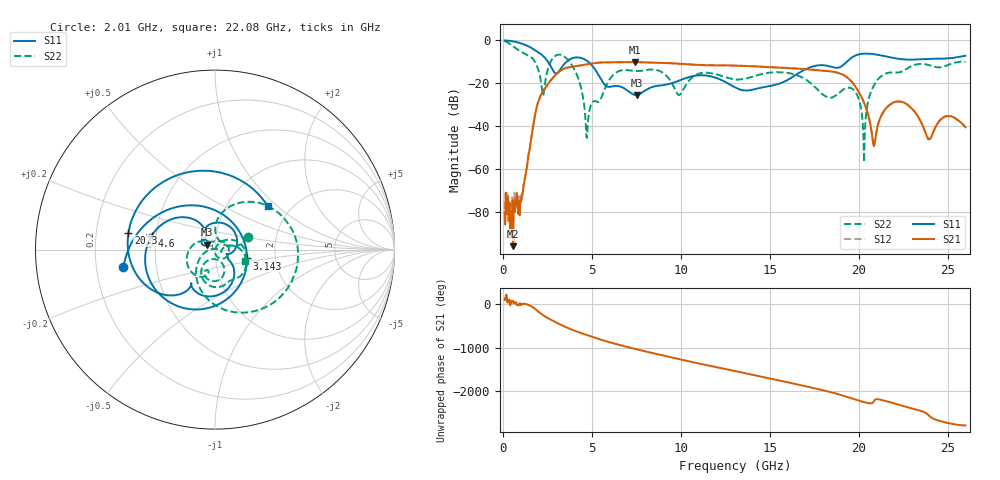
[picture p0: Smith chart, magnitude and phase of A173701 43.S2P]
!  2-Port S-parameters saved by WinCal
! VAR MeasName=S-Parameters (CALIBRATED_DATA) read from VNA (N5245A)
! VAR MeasDate=2017-6-7 10:31:17
! VAR NAME=A173701 43
! VAR FILENAME=A173701 43.S2P
! VAR DATE=2017-6-7 10:31:17
! VAR PHYS_PORTS=1,2
# Hz S DB R 50
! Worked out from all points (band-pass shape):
!   801 points, 100 MHz to 26 GHz, reference 50 ohm
!   highest |S21| = -10.12 dB at 7.417 GHz (marker M1); lowest = -96.1 dB at 585.6 MHz (marker M2)
!   |S21| within 3 dB of the highest: 3.466 GHz to 16.34 GHz (12.88 GHz wide, 130 % of centre); 16.35897 GHz to 16.39744 GHz (38.47 MHz wide, 0.235 % of centre)
!   lowest |S11| = -25.5 dB at 7.514 GHz (marker M3), VSWR 1.11, Z = 45.6 + j2.53 ohm
!   |S11| at or under -10 dB: 2.54 GHz to 3.573 GHz (1.033 GHz wide, 33.8 % of centre); 4.804 GHz to 19.33 GHz (14.52 GHz wide, 120 % of centre)
!   |S22| runs from -56.9 to -0.2 dB; largest |S21 - S12| = 0.0047
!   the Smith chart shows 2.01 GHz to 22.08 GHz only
!   S11 on the Smith chart (normalised r, x): 2.01 GHz: 0.32, -0.09; 3.143 GHz: 1.43, -0.15; 4.6 GHz: 0.47, +0.09; 20.3 GHz: 0.34, +0.08; 22.08 GHz: 1.53, +0.87
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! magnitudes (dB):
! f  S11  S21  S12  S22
! 100 MHz  0.0  -80.5  -75.4  -0.2
! 585.6 MHz  -0.5  -96.1  -76.2  -2.8
! 1.071 GHz  -1.5  -71.9  -74.6  -5.5
! 2.01 GHz  -5.7  -28.2  -28.2  -14.2
! 2.269 GHz  -7.3  -23.7  -23.7  -25.7
! 3.143 GHz  -14.6  -14.7  -14.7  -6.6
! 4.438 GHz  -8.3  -11.6  -11.6  -23.6
! 4.6 GHz  -8.9  -11.4  -11.4  -32.3
! 7.417 GHz  -25.4  -10.1  -10.1  -14.3
! 7.514 GHz  -25.5  -10.1  -10.2  -14.3
! 8.744 GHz  -21.1  -10.4  -10.5  -14.1
! 9.91 GHz  -18.8  -10.9  -10.9  -25.5
! 13.05 GHz  -21.9  -11.8  -11.8  -18.3
! 17.39 GHz  -12.2  -13.7  -13.6  -20.6
! 19.69 GHz  -7.6  -20.0  -20.0  -22.8
! 20.3 GHz  -6.2  -29.0  -29.1  -56.9
! 20.85 GHz  -6.4  -49.4  -49.7  -21.1
! 21.69 GHz  -7.7  -30.4  -30.6  -15.1
! 22.08 GHz  -8.4  -28.6  -28.8  -15.0
! 23.96 GHz  -8.6  -46.2  -46.1  -11.5
! 24.87 GHz  -8.5  -35.6  -35.4  -12.0
! 26 GHz  -7.2  -40.6  -40.4  -10.0
